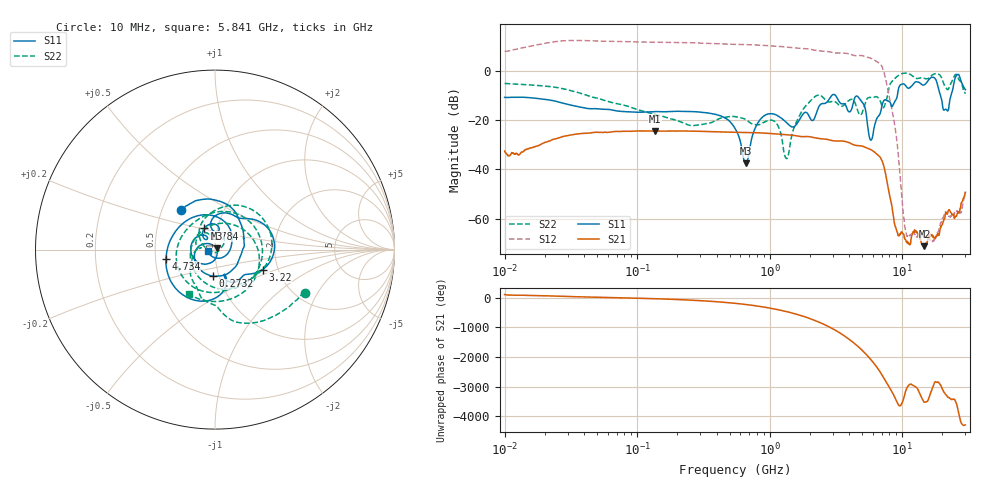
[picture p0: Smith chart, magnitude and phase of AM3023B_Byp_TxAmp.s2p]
# Hz S DB R 50.0
!freq dBS11 angS11 dBS21 angS21 dBS12 angS12 dBS22 angS22
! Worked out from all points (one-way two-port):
!   1601 points, 10 MHz to 30 GHz, reference 50 ohm
!   highest |S21| = -24.34 dB at 135.6 MHz (marker M1); lowest = -71.2 dB at 14.74 GHz (marker M2)
!   lowest |S11| = -37.5 dB at 659.1 MHz (marker M3), VSWR 1.03, Z = 51.2 + j0.651 ohm
!   |S11| at or under -10 dB: start of sweep to 2.942 GHz; 3.143 GHz to 9.198 GHz (6.055 GHz wide, 98.1 % of centre); 19.49 GHz to 23.37 GHz (3.88 GHz wide, 18.1 % of centre)
!   |S22| runs from -35.6 to -0.9 dB; largest |S21 - S12| = 4.2
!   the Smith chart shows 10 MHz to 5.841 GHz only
!   S11 on the Smith chart (normalised r, x): 10 MHz: 0.62, +0.30; 273.2 MHz: 0.93, -0.28; 1.784 GHz: 0.86, +0.21; 3.22 GHz: 1.66, -0.40; 4.734 GHz: 0.57, -0.06; 5.841 GHz: 0.93, -0.02
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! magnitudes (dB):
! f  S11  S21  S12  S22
! 10 MHz  -10.8  -32.5  7.9  -5.1
! 38.04 MHz  -14.8  -25.4  12.3  -9.2
! 135.6 MHz  -16.5  -24.3  11.6  -17.7
! 144.7 MHz  -16.5  -24.4  11.6  -18.0
! 273.2 MHz  -16.6  -24.5  11.4  -22.1
! 547.7 MHz  -23.3  -24.9  10.8  -18.6
! 659.1 MHz  -37.5  -25.0  10.6  -19.7
! 876.7 MHz  -18.9  -25.2  10.4  -21.3
! 1.126 GHz  -17.9  -25.6  10.0  -21.3
! 1.341 GHz  -21.0  -25.9  9.7  -35.6
! 1.784 GHz  -17.6  -26.7  9.1  -15.7
! 2.084 GHz  -20.1  -26.9  8.6  -11.6
! 3.22 GHz  -10.8  -28.5  7.2  -13.1
! 4.734 GHz  -11.1  -30.3  6.3  -17.5
! 5.841 GHz  -28.1  -32.0  5.1  -10.8
! 7.926 GHz  -12.4  -48.9  -9.4  -7.1
! 10.7 GHz  -6.2  -69.1  -65.9  -0.9
! 14.74 GHz  -5.6  -71.2  -67.5  -3.1
! 17.56 GHz  -2.9  -68.1  -67.7  -1.2
! 21.35 GHz  -15.6  -57.4  -57.2  -6.8
! 25.82 GHz  -1.7  -58.6  -56.9  -1.5
! 30 GHz  -7.6  -49.4  -49.0  -9.3
